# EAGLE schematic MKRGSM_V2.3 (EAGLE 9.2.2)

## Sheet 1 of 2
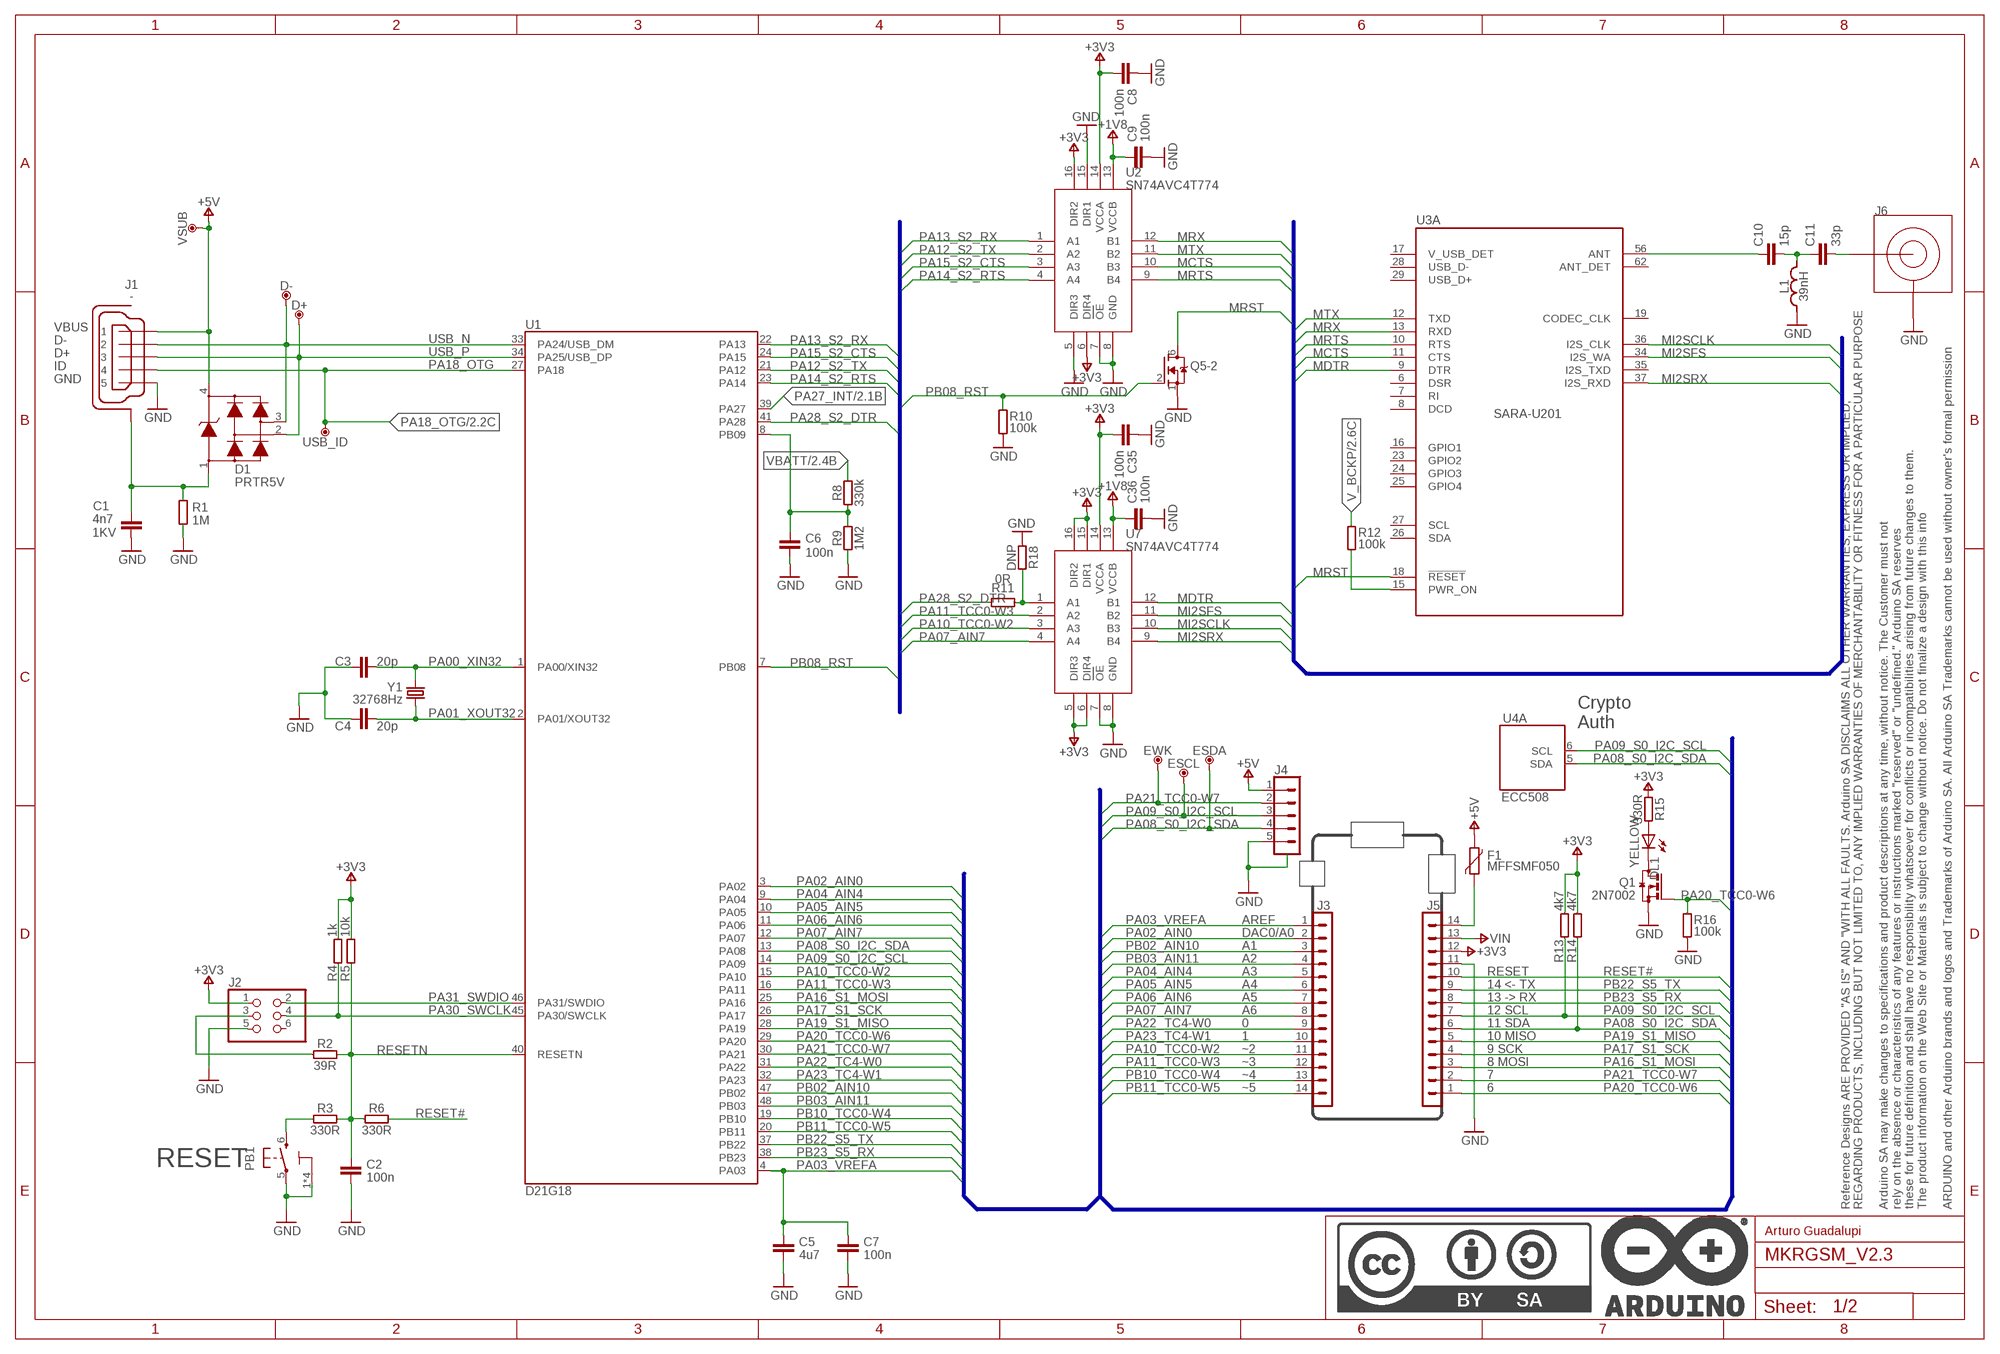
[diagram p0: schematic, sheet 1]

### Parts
C1  4n7  C4.7NF-0805  [0805-R2013X50N]
C2  100n  C-100NF-0402  [0402-1005X55N]
C3  20p  C-20PF-0402  [0402-1005X55N]
C4  20p  C-20PF-0402  [0402-1005X55N]
C5  4u7  C-4.7UF-0402  [0402-1005X55N]
C6  100n  C-100NF-0402  [0402-1005X55N]
C7  100n  C-100NF-0402  [0402-1005X55N]
C8  100n  C-100NF-0402  [0402-1005X55N]
C9  100n  C-100NF-0402  [0402-1005X55N]
C10  15p  C-15PF-0402  [0402-1005X55N]
C11  33p  C-33PF-0402  [0402-1005X55N]
C35  100n  C-100NF-0402  [0402-1005X55N]
C36  100n  C-100NF-0402  [0402-1005X55N]
D1  PRTR5V  PRTR5V0U2X,215  [SOT190P230X110-4N]
D+  DNP  TPTP-1.00MM  [TP-1.00MM]
D-  DNP  TPTP-1.00MM  [TP-1.00MM]
DL1  YELLOW  LED-YELLOW-0603  [LEDC1608X80N-AK]
ESCL  DNP  TPTP-1.00MM  [TP-1.00MM]
ESDA  DNP  TPTP-1.00MM  [TP-1.00MM]
EWK  DNP  TPTP-1.00MM  [TP-1.00MM]
F1  MFFSMF050  PTC  [0603-1608X90N]
FRAME1  DNP  A3-FRAME  [FRAME]
J1  -  USB-MICRO  [ZX62-AB-5PA]
J2  DNP  PINHD-2X03-DNPSMD-NH  [2X3_SMT]
J3  -  PINHD-1X14-SM-MALE/FEMALETH-SMD  [1X14_SMD_TH]
J4  -  SM05B-SRSS-TB  [SM05B-SRSS-TB]
J5  -  PINHD-1X14-SM-MALE/FEMALETH-SMD  [1X14_SMD_TH]
J6  -  UFL  [U.FL-R-SMT-1(60)]
L1  39nH  L-39NH-0402  [C0402]
PB1  PTS820  TACTILE1PTS820-NH  [C&K_PTS820_NO_HOLES]
Q1  2N7002  2N7002T  [SOTFL50P160X78-3]
Q5  2N7002DW-7-FNO_PAD  [PWR_SC70-6L2]
R1  1M  R-1M-0402  [0402-1005X55N]
R2  39R  R-39R-0402  [0402-1005X55N]
R3  330R  R-330R-0402  [0402-1005X55N]
R4  1k  R-1K-0402  [0402-1005X55N]
R5  10k  R-10K-0402  [0402-1005X55N]
R6  330R  R-330R-0402  [0402-1005X55N]
R8  330k  R-330K-0402  [0402-1005X55N]
R9  1M2  R-1M2-0402  [0402-1005X55N]
R10  100k  R-100K-0402  [0402-1005X55N]
R11  0R  R-0R-0402  [0402-1005X55N]
R12  100k  R-100K-0402  [0402-1005X55N]
R13  4k7  R-4K7-0402  [0402-1005X55N]
R14  4k7  R-4K7-0402  [0402-1005X55N]
R15  330R  R-330R-0402  [0402-1005X55N]
R16  100k  R-100K-0402  [0402-1005X55N]
R18  DNP  R-DNP-0402  [0402-1005X55N]
U1  D21G18  ATSAMD21G18A-48QFN  [QFN50P700X700X90-49XN-EPSQ515]
U2  SN74AVC4T774  [RSV]
U3  SARA-U201  SARA-U2  [SARA-96]
U4  ECC508  ATECC508A-MAHDA-T8-UDFN  [SON50P300X200X60-9N-EP160X140]
U7  SN74AVC4T774  [RSV]
USB_ID  DNP  TPTP-1.00MM  [TP-1.00MM]
VSUB  DNP  TPTP-1.00MM  [TP-1.00MM]
Y1  32768Hz  32.768KHZ  [ABS07]

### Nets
+1V8: C9.1 C36.1 U2.13(VCCB) U7.13(VCCB) ; also sheet 2
+3V3: C8.2 C35.2 J2.1 J5.12 R4.2 R5.2 R13.2 R14.2 R15.1 U2.6(DIR4) U2.14(VCCA) U2.16(DIR2) U7.5(DIR3) U7.6(DIR4) U7.14(VCCA) U7.15(DIR1) U7.16(DIR2) ; also sheet 2
+5V: D1.4 F1.2 J1.1 J4.1 VSUB.X ; also sheet 2
GND: C1.2 C2.2 C3.1 C4.1 C5.2 C6.2 C7.2 C8.1 C9.2 C35.1 C36.2 J1.5 J2.5 J4.5 J4.SH1(SH) J4.SH2(SH) J5.11 J6.GND1(GND) J6.GND2(GND) L1.1 PB1.1 PB1.2 PB1.3 PB1.4 PB1.5 Q1.S Q5.1(-2:S) R1.1 R9.1 R10.1 R16.1 R18.1 U2.5(DIR3) U2.7(OE) U2.8(GND) U2.15(DIR1) U7.7(OE) U7.8(GND) ; also sheet 2
MCTS: U2.10(B3) U3.11(A:CTS)
MDTR: U3.9(A:DTR) U7.12(B1)
MI2SCLK: U3.36(A:I2S_CLK) U7.10(B3)
MI2SFS: U3.34(A:I2S_WA) U7.11(B2)
MI2SRX: U3.37(A:I2S_RXD) U7.9(B4)
MRST: Q5.6(-2:D) U3.18(A:!RESET)
MRTS: U2.9(B4) U3.10(A:RTS)
MRX: U2.12(B1) U3.13(A:RXD)
MTX: U2.11(B2) U3.12(A:TXD)
N17658775: PB1.6 R3.1
N$1: C1.1 D1.1 J1.6(SH) J1.7(SH) J1.8(SH) J1.9(SH) J1.10(SH) J1.11(SH) R1.2
N$2: F1.1 J5.14
N$4: J2.3 R2.1
N$5: C10.1 U3.56(A:ANT)
N$6: C6.1 R8.1 R9.2 U1.8(PB09)
N$7: DL1.A R15.2
N$8: C11.2 J6.SIG
N$9: R11.1 R18.2 U7.1(A1)
N$10: DL1.C Q1.D
N$13: R12.1 U3.15(A:PWR_ON)
N$14: C10.2 C11.1 L1.2
PA00_XIN32: C3.2 U1.1(PA00/XIN32) Y1.2
PA01_XOUT32: C4.2 U1.2(PA01/XOUT32) Y1.1
PA02_AIN0: J3.2 U1.3(PA02)
PA03_VREFA: C5.1 C7.1 J3.1 U1.4(PA03)
PA04_AIN4: J3.5 U1.9(PA04)
PA05_AIN5: J3.6 U1.10(PA05)
PA06_AIN6: J3.7 U1.11(PA06)
PA07_AIN7: J3.8 U1.12(PA07) U7.4(A4)
PA08_S0_I2C_SDA: ESDA.X J4.4 J5.6 R14.1 U1.13(PA08) U4.5(A:SDA) ; also sheet 2
PA09_S0_I2C_SCL: ESCL.X J4.3 J5.7 R13.1 U1.14(PA09) U4.6(A:SCL) ; also sheet 2
PA10_TCC0-W2: J3.11 U1.15(PA10) U7.3(A3)
PA11_TCC0-W3: J3.12 U1.16(PA11) U7.2(A2)
PA12_S2_TX: U1.21(PA12) U2.2(A2)
PA13_S2_RX: U1.22(PA13) U2.1(A1)
PA14_S2_RTS: U1.23(PA14) U2.4(A4)
PA15_S2_CTS: U1.24(PA15) U2.3(A3)
PA16_S1_MOSI: J5.3 U1.25(PA16)
PA17_S1_SCK: J5.4 U1.26(PA17)
PA18_OTG: J1.4 U1.27(PA18) USB_ID.X ; also sheet 2
PA19_S1_MISO: J5.5 U1.28(PA19)
PA20_TCC0-W6: J5.1 Q1.G R16.2 U1.29(PA20)
PA21_TCC0-W7: EWK.X J4.2 J5.2 U1.30(PA21)
PA22_TC4-W0: J3.9 U1.31(PA22)
PA23_TC4-W1: J3.10 U1.32(PA23)
PA27_INT: U1.39(PA27) ; also sheet 2
PA28_S2_DTR: R11.2 U1.41(PA28)
PA30_SWCLK: J2.4 R4.1 U1.45(PA30/SWCLK)
PA31_SWDIO: J2.2 U1.46(PA31/SWDIO)
PB02_AIN10: J3.3 U1.47(PB02)
PB03_AIN11: J3.4 U1.48(PB03)
PB08_RST: Q5.2(-2:G) R10.2 U1.7(PB08)
PB10_TCC0-W4: J3.13 U1.19(PB10)
PB11_TCC0-W5: J3.14 U1.20(PB11)
PB22_S5_TX: J5.9 U1.37(PB22)
PB23_S5_RX: J5.8 U1.38(PB23)
RESET#: J5.10 R6.2
RESETN: C2.1 R2.2 R3.2 R5.1 R6.1 U1.40(RESETN)
USB_N [usb]: D1.3 D-.X J1.2 U1.33(PA24/USB_DM) ; also sheet 2
USB_P [usb]: D1.2 D+.X J1.3 U1.34(PA25/USB_DP) ; also sheet 2
V_BCKP: R12.2 ; also sheet 2
VBATT: R8.2 ; also sheet 2
VIN: J5.13 ; also sheet 2
Unconnected: J2.6 U3.6(A:DSR) U3.7(A:RI) U3.8(A:DCD) U3.16(A:GPIO1) U3.17(A:V_USB_DET) U3.19(A:CODEC_CLK) U3.23(A:GPIO2) U3.24(A:GPIO3) U3.25(A:GPIO4) U3.26(A:SDA) U3.27(A:SCL) U3.28(A:USB_D-) U3.29(A:USB_D+) U3.35(A:I2S_TXD) U3.62(A:ANT_DET)

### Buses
PA03_VREFA,PA02_AIN0,PB02_AIN10,PB03_AIN11,PA04_AIN4,PA05_AIN5,PA06_AIN6,PA07_AIN7,PA22_TC4-W0,PA23_TC4-W1,PA10_TCC0-W2,PA11_TCC0-W3,PB10_TCC0-W4,PB11_TCC0-W5,PA20_TCC0-W6,PA21_TCC0-W7,PA16_S1_MOSI,PA17_S1_SCK,PA19_S1_MISO,PA08_S0_I2C_SDA,PA09_S0_I2C_SCL,PB23_S5_RX,PB22_S5_TX,RESET#
MI2SCLK
B$2

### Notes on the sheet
- Crypto
  Auth
- AREF
- DAC0/A0
- A1
- A2
- A3 | RESET
- A4 | 14 <- TX
- A5 | 13 -> RX
- A6 | 12 SCL
- 0 | 11 SDA
- 1 | 10 MISO
- ~2 | 9 SCK
- ~3 | 8 MOSI
- ~4 | 7
- ~5 | 6
- RESET
- Arturo Guadalupi

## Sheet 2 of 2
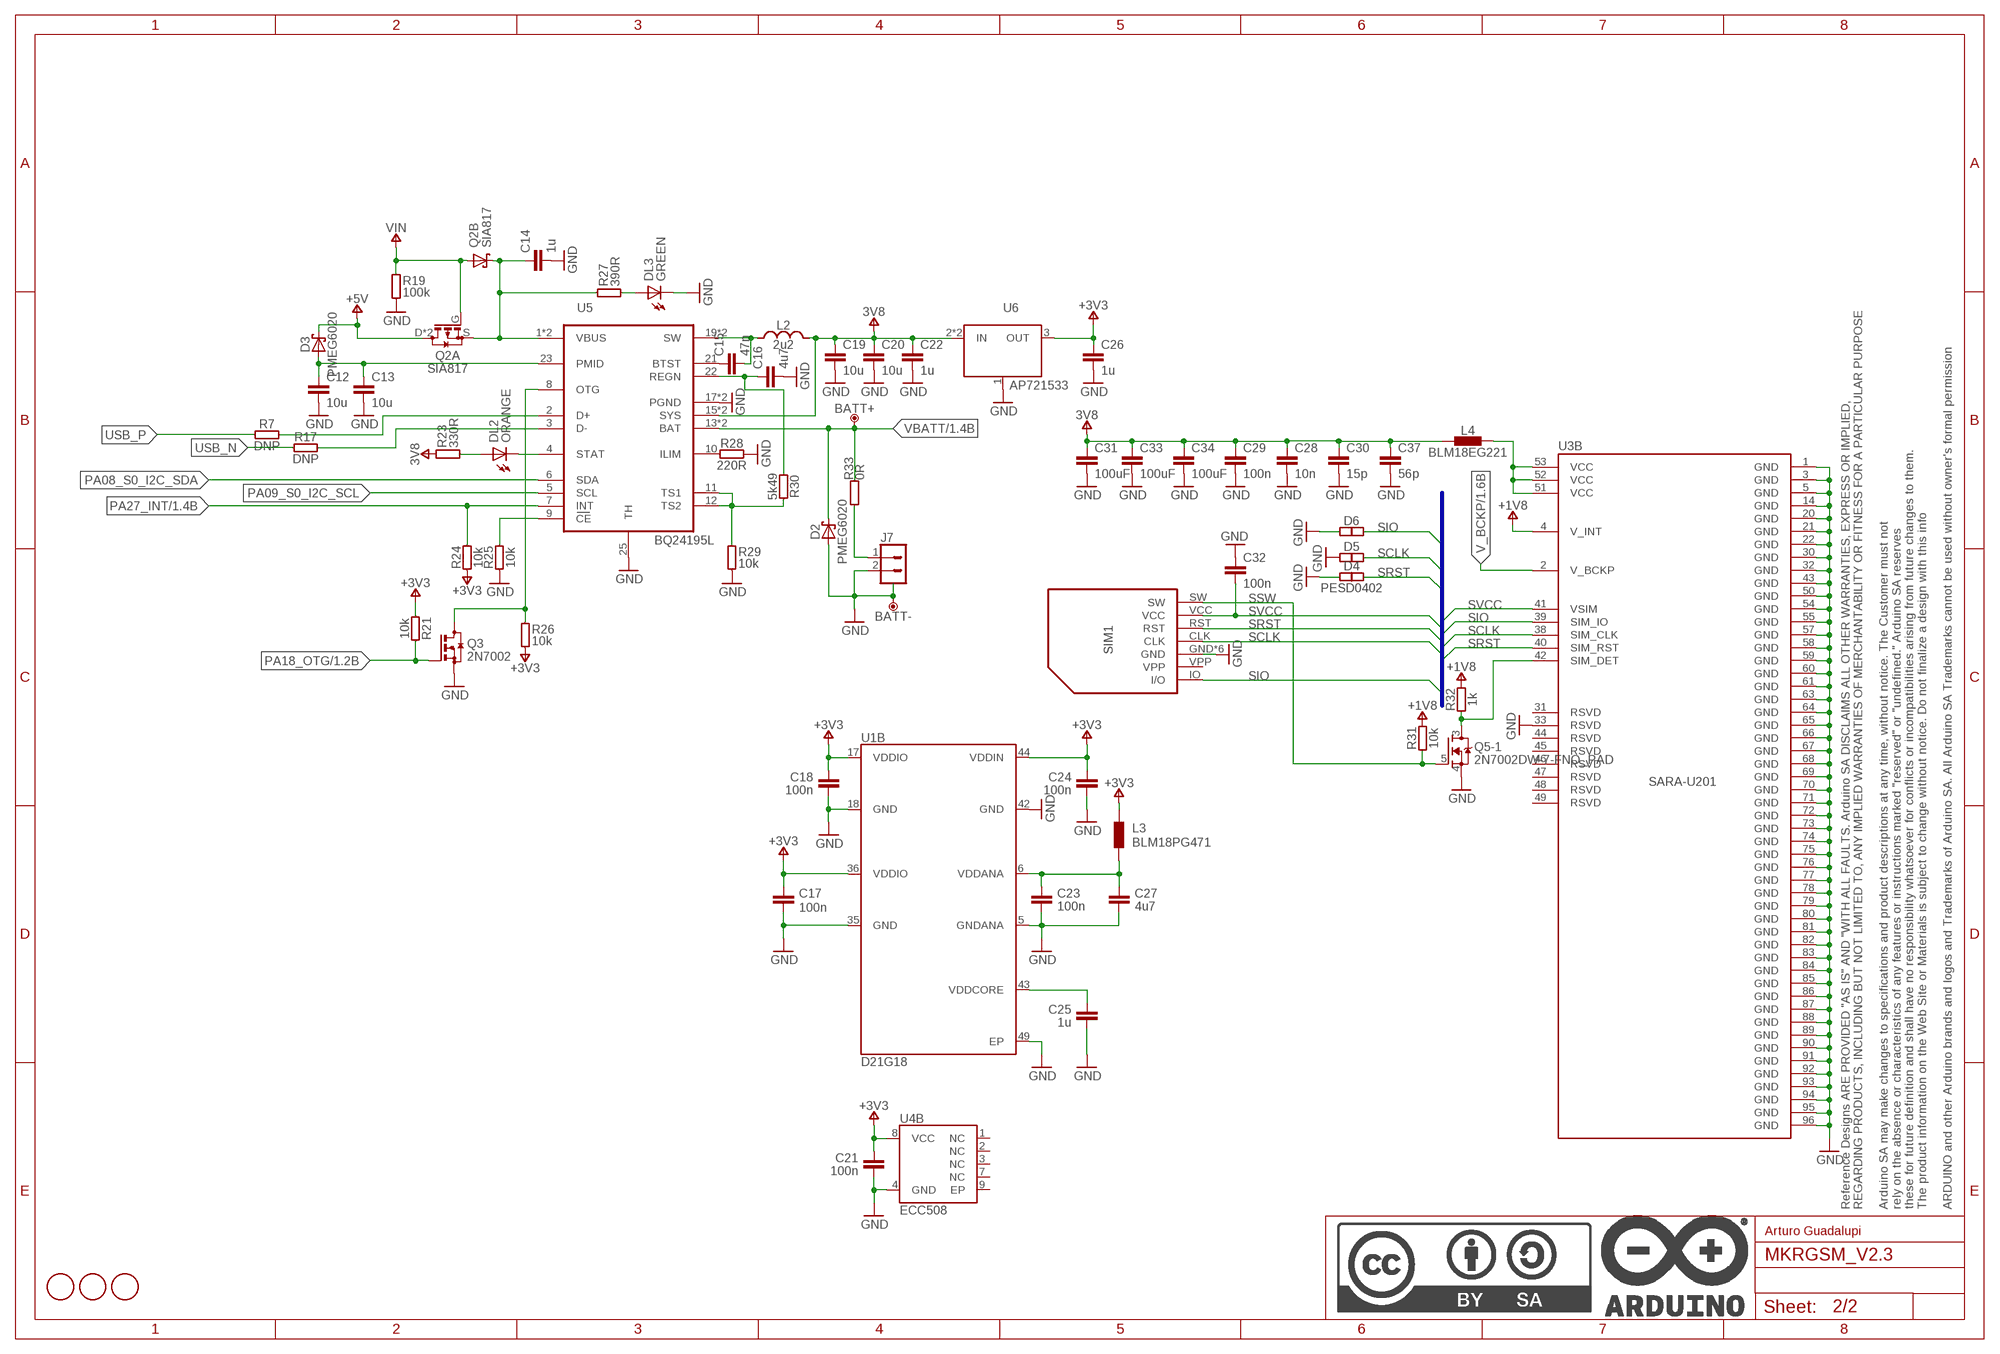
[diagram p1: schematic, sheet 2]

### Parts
BATT+  DNP  TPTP-1.00MM  [TP-1.00MM]
BATT-  DNP  TPTP-1.00MM  [TP-1.00MM]
C12  10u  C-10UF-0603  [0603-1608X90N]
C13  10u  C-10UF-0603  [0603-1608X90N]
C14  1u  C-1UF-0402  [0402-1005X55N]
C15  47n  C-47N-0402  [0402-1005X55N]
C16  4u7  C-4.7UF-0402  [0402-1005X55N]
C17  100n  C-100NF-0402  [0402-1005X55N]
C18  100n  C-100NF-0402  [0402-1005X55N]
C19  10u  C-10UF-0603  [0603-1608X90N]
C20  10u  C-10UF-0603  [0603-1608X90N]
C21  100n  C-100NF-0402  [0402-1005X55N]
C22  1u  C-1UF-0402  [0402-1005X55N]
C23  100n  C-100NF-0402  [0402-1005X55N]
C24  100n  C-100NF-0402  [0402-1005X55N]
C25  1u  C-1UF-0402  [0402-1005X55N]
C26  1u  C-1UF-0402  [0402-1005X55N]
C27  4u7  C-4.7UF-0603  [0603-1608X90N]
C28  10n  C-10NF-0402  [0402-1005X55N]
C29  100n  C-100NF-0402  [0402-1005X55N]
C30  15p  C-15PF-0402  [0402-1005X55N]
C31  100uF  C-100UF-1206  [C1206]
C32  100n  C-100NF-0402  [0402-1005X55N]
C33  100uF  C-100UF-1206  [C1206]
C34  100uF  C-100UF-1206  [C1206]
C37  56p  C-56P-0402  [0402-1005X55N]
D2  PMEG6020  PMEG6020AELRX  [SODFL3517X110N]
D3  PMEG6020  PMEG6020AELRX  [SODFL3517X110N]
D4  PESD0402  PESD  [0402-1005X55N]
D5  PESD0402  PESD  [0402-1005X55N]
D6  PESD0402  PESD  [0402-1005X55N]
DL2  ORANGE  LED-ORANGE-0603  [LEDC1608X80N-AK]
DL3  GREEN  LED-GREEN-0603  [LEDC1608X80N-AK]
FD1  DNP  FIDUCIAL-1.5MM  [FD-1-1.5]
FD2  DNP  FIDUCIAL-1.5MM  [FD-1-1.5]
FD3  DNP  FIDUCIAL-1.5MM  [FD-1-1.5]
FRAME2  DNP  A3-FRAME  [FRAME]
J7  -  BATTERY  [JST-S2B-PH-SM4-TB]
L2  2u2  LSRP  [SRP4020]
L3  BLM18PG471  FERRITE-470R  [0603-1608X90N]
L4  BLM18EG221  FERRITE-220R  [0603-1608X90N]
Q2  SIA817  SIA817EDJ  [SON65P205X205X75-8N-MWSD]
Q3  2N7002  2N7002T  [SOTFL50P160X78-3]
R7  DNP  R-DNP-0402  [0402-1005X55N]
R17  DNP  R-DNP-0402  [0402-1005X55N]
R19  100k  R-100K-0402  [0402-1005X55N]
R21  10k  R-10K-0402  [0402-1005X55N]
R23  330R  R-330R-0402  [0402-1005X55N]
R24  10k  R-10K-0402  [0402-1005X55N]
R25  10k  R-10K-0402  [0402-1005X55N]
R26  10k  R-10K-0402  [0402-1005X55N]
R27  390R  R-390R-0402  [0402-1005X55N]
R28  220R  R-220R-0402  [0402-1005X55N]
R29  10k  R-10K-0402  [0402-1005X55N]
R30  5k49  R-5K49-0402  [0402-1005X55N]
R31  10k  R-10K-0402  [0402-1005X55N]
R32  1k  R-1K-0402  [0402-1005X55N]
R33  0R  R-0R-0603  [C0603]
SIM1  -  SIM  [MICROSIM8]
U5  BQ24195L  BQ24195QFN-24  [QFN24]
U6  AP721533  AP7215-33YG  [SOT89-3L]

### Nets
+1V8: R31.2 R32.2 U3.4(B:V_INT) ; also sheet 1
+3V3: C17.1 C18.1 C21.1 C24.1 C26.1 L3.1 R21.1 R24.1 R26.1 U1.17(VDDIO) U1.36(VDDIO) U1.44(VDDIN) U4.8(B:VCC) U6.3(OUT) ; also sheet 1
+3V8: C19.1 C20.1 C22.1 C28.1 C29.1 C30.1 C31.1 C33.1 C34.1 C37.1 L2.2 L4.1 R23.2 U5.15(SYS) U5.16(SYS) U6.2(IN) U6.TH(IN) ; supply symbol labelled 3V8
+5V: D3.C Q2.D2(A:D) Q2.D(A:D) ; also sheet 1
GND: BATT-.X C12.2 C13.2 C14.2 C16.2 C17.2 C18.2 C19.2 C20.2 C21.2 C22.2 C23.2 C24.2 C25.2 C26.2 C27.2 C28.2 C29.2 C30.2 C31.2 C32.1 C33.2 C34.2 C37.2 D2.A D4.1 D5.1 D6.1 DL3.C J7.2 J7.3(SH) J7.4(SH) Q3.S Q5.4(-1:S) R19.1 R25.1 R28.2 R29.1 SIM1.GND SIM1.SH1(GND) SIM1.SH2(GND) SIM1.SH3(GND) SIM1.SH4(GND) SIM1.SH5(GND) U1.5(GNDANA) U1.18(GND) U1.35(GND) U1.42(GND) U1.49(EP) U3.1(B:GND) U3.3(B:GND) U3.5(B:GND) U3.14(B:GND) U3.20(B:GND) U3.21(B:GND) U3.22(B:GND) U3.30(B:GND) U3.32(B:GND) U3.33(B:RSVD) U3.43(B:GND) U3.50(B:GND) U3.54(B:GND) U3.55(B:GND) U3.57(B:GND) U3.58(B:GND) U3.59(B:GND) U3.60(B:GND) U3.61(B:GND) U3.63(B:GND) U3.64(B:GND) U3.65(B:GND) U3.66(B:GND) U3.67(B:GND) U3.68(B:GND) U3.69(B:GND) U3.70(B:GND) U3.71(B:GND) U3.72(B:GND) U3.73(B:GND) U3.74(B:GND) U3.75(B:GND) U3.76(B:GND) U3.77(B:GND) U3.78(B:GND) U3.79(B:GND) U3.80(B:GND) U3.81(B:GND) U3.82(B:GND) U3.83(B:GND) U3.84(B:GND) U3.85(B:GND) U3.86(B:GND) U3.87(B:GND) U3.88(B:GND) U3.89(B:GND) U3.90(B:GND) U3.91(B:GND) U3.92(B:GND) U3.93(B:GND) U3.94(B:GND) U3.95(B:GND) U3.96(B:GND) U4.4(B:GND) U5.17(PGND) U5.18(PGND) U5.25(TH) U6.1(GND/ADJ) ; also sheet 1
N17798864: DL2.A R23.1
N17834267: DL3.A R27.1
N17852357: C23.1 C27.1 L3.2 U1.6(VDDANA)
N17852431: C25.1 U1.43(VDDCORE)
N$3: J7.1 R33.1
N$11: Q5.3(-1:D) R32.1 U3.42(B:SIM_DET)
N$12: L4.2 U3.51(B:VCC) U3.52(B:VCC) U3.53(B:VCC)
N$15: C15.2 L2.1 U5.19(SW) U5.20(SW)
N$16: R7.2 U5.2(D+)
N$17: C14.1 Q2.K2(B:C) Q2.K(B:C) Q2.S(A:S) R27.2 U5.1(VBUS) U5.24(VBUS)
N$18: C15.1 U5.21(BTST)
N$19: R28.1 U5.10(ILIM)
N$20: R17.2 U5.3(D-)
N$21: C16.1 R30.1 U5.22(REGN)
N$22: Q3.D R26.2 U5.8(OTG)
N$23: R29.2 R30.2 U5.11(TS1) U5.12(TS2)
N$24: R25.2 U5.9(CE)
PA08_S0_I2C_SDA: U5.6(SDA) ; also sheet 1
PA09_S0_I2C_SCL: U5.5(SCL) ; also sheet 1
PA18_OTG: Q3.G R21.2 ; also sheet 1
PA27_INT: R24.2 U5.7(INT) ; also sheet 1
SCLK: D5.2 SIM1.CLK U3.38(B:SIM_CLK)
SIO: D6.2 SIM1.IO(I/O) U3.39(B:SIM_IO)
SRST: D4.2 SIM1.RST U3.40(B:SIM_RST)
SSW: Q5.5(-1:G) R31.1 SIM1.SW
STAT: DL2.C U5.4(STAT)
SVCC: C32.2 SIM1.VCC U3.41(B:VSIM)
USB_N [usb]: R17.1 ; also sheet 1
USB_P [usb]: R7.1 ; also sheet 1
V_BCKP: U3.2(B:V_BCKP) ; also sheet 1
VBATT: BATT+.X D2.C R33.2 U5.13(BAT) U5.14(BAT) ; also sheet 1
VIN: Q2.A(B:A) Q2.G(A:G) R19.2 ; also sheet 1
VUSB1: C12.1 C13.1 D3.A U5.23(PMID)
Unconnected: SIM1.VPP U3.31(B:RSVD) U3.44(B:RSVD) U3.45(B:RSVD) U3.46(B:RSVD) U3.47(B:RSVD) U3.48(B:RSVD) U3.49(B:RSVD) U4.1(B:NC) U4.2(B:NC) U4.3(B:NC) U4.7(B:NC) U4.9(B:EP)

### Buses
B$1

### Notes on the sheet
- Arturo Guadalupi

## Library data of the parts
BATT+ BATT- D+ D- ESCL ESDA EWK USB_ID VSUB = Arduino-utility:TP: Testpoint; DATASHEET: DNP; DISTRIBUTOR-LINK: DNP; DISTRIBUTOR-PN: DNP; MANUFACTURER: DNP; MANUFACTURER-PN: DNP
C1 = Arduino-rcl:C: SMD Capacitor; CODE-ARDUINO: 0689; DATASHEET: http://www.kemet.com/Lists/ProductCatalog/Attachments/40/KEM_C1010_X7R_HV_SMD.pdf; DISTRIBUTOR-LINK: www.kemet.com/docfinder?Partnumber=C0805C472KDRACTU; DISTRIBUTOR-PN: 399-6738-1-ND; MANUFACTURER: Kemet; MANUFACTURER-PN: C0805C472KDRACTU; NOTE: -; VOLTAGE: 1KV
C2 C6-C9 C17 C18 C21 C23 C24 C29 C32 C35 C36 = Arduino-rcl:C: SMD Capacitor; CODE-ARDUINO: 0132; DATASHEET: http://www.tdk.com/pdf/TDKMLCCCapRange.pdf; DISTRIBUTOR-LINK: http://www.digikey.com/product-detail/en/tdk-corporation/C1005X5R1H104K050BB/445-5942-1-ND/2443982; DISTRIBUTOR-PN: 445-5942-1-ND; MANUFACTURER: TDK; MANUFACTURER-PN: C1005X5R1H104K050BB; NOTE: -
C3 C4 = Arduino-rcl:C: SMD Capacitor; CODE-ARDUINO: 2188; DATASHEET: http://www.kemet.com/docfinder?Partnumber=CBR04C200J5GAC; DISTRIBUTOR-LINK: http://www.digikey.com/product-detail/en/kemet/CBR04C200J5GAC/399-6173-1-ND/2732143; DISTRIBUTOR-PN: 399-6173-1-ND; MANUFACTURER: Kemet; MANUFACTURER-PN: CBR04C200J5GAC; NOTE: -
C5 C16 = Arduino-rcl:C: SMD Capacitor; CODE-ARDUINO: 0833; DATASHEET: http://search.murata.co.jp/Ceramy/image/img/A01X/partnumbering_e_01.pdf; DISTRIBUTOR-LINK: http://www.digikey.com/product-detail/en/murata-electronics-north-america/GRM155R60J475ME47D/490-5915-1-ND/3719860; DISTRIBUTOR-PN: 490-5915-1-ND; MANUFACTURER: Murata; MANUFACTURER-PN: GRM155R60J475ME47D; NOTE: -
C10 C30 = Arduino-rcl:C: SMD Capacitor; CODE-ARDUINO: -; DATASHEET: http://search.murata.co.jp/Ceramy/image/img/A01X/partnumbering_e_01.pdf; DISTRIBUTOR-LINK: https://www.digikey.com/product-detail/en/murata-electronics-north-america/GRM1555C1H150JA01D/490-5888-1-ND/3315234; DISTRIBUTOR-PN: 490-5888-1-ND; MANUFACTURER: Murata; MANUFACTURER-PN: GRM1555C1H150JA01D; NOTE: -
C11 = Arduino-rcl:C: SMD Capacitor; CODE-ARDUINO: -; DATASHEET: http://www.murata.com/~/media/webrenewal/support/library/catalog/products/capacitor/mlcc/c02e.pdf; DISTRIBUTOR-LINK: http://www.digikey.com/product-search/en?keywords=490-5936-1-ND; DISTRIBUTOR-PN: 490-5936-1-ND; MANUFACTURER: Murata; MANUFACTURER-PN: GRM1555C1H330JA01D; NOTE: -
C12 C13 C19 C20 = Arduino-rcl:C: SMD Capacitor; CODE-ARDUINO: 2213; DATASHEET: http://www.murata.com/~/media/webrenewal/support/library/catalog/products/capacitor/mlcc/c02e.pdf; DISTRIBUTOR-LINK: http://www.digikey.com/product-search/en?keywords=490-10728-1-ND; DISTRIBUTOR-PN: 490-10728-1-ND; MANUFACTURER: Murata; MANUFACTURER-PN: GRM188R61C106KAALD; NOTE: -
C14 C22 C25 C26 = Arduino-rcl:C: SMD Capacitor; CODE-ARDUINO: 0133; DATASHEET: http://search.murata.co.jp/Ceramy/image/img/A01X/partnumbering_e_01.pdf; DISTRIBUTOR-LINK: http://www.digikey.com/product-detail/en/murata-electronics-north-america/GRM155R61E105KA12D/490-10017-1-ND/5026367; DISTRIBUTOR-PN: 490-10017-1-ND; MANUFACTURER: Murata; MANUFACTURER-PN: GRM155R61E105KA12D; NOTE: -
C15 = Arduino-rcl:C: SMD Capacitor; CODE-ARDUINO: 2216; DATASHEET: http://www.murata.com/~/media/webrenewal/support/library/catalog/products/capacitor/mlcc/c02e.pdf; DISTRIBUTOR-LINK: https://www.digikey.com/product-detail/en/murata-electronics-north-america/GRM155R71E473KA88D/490-3254-1-ND/702795; DISTRIBUTOR-PN: 490-3254-1-ND; MANUFACTURER: Murata; MANUFACTURER-PN: GRM155R71E473KA88D; NOTE: -
C27 = Arduino-rcl:C: SMD Capacitor; CODE-ARDUINO: 0458; DATASHEET: http://www.murata.com/~/media/webrenewal/support/library/catalog/products/capacitor/mlcc/c02e.pdf; DISTRIBUTOR-LINK: http://www.digikey.com/product-search/en?keywords=490-7203-1-ND; DISTRIBUTOR-PN: 490-7203-1-ND; MANUFACTURER: Murata; MANUFACTURER-PN: GRM188R61E475KE11D; NOTE: -
C28 = Arduino-rcl:C: SMD Capacitor; CODE-ARDUINO: 0165; DATASHEET: http://search.murata.co.jp/Ceramy/image/img/A01X/partnumbering_e_01.pdf; DISTRIBUTOR-LINK: http://www.digikey.com/product-detail/en/murata-electronics-north-america/GRM155R71H103KA88J/490-6351-1-ND/3845548; DISTRIBUTOR-PN: 490-6351-1-ND; MANUFACTURER: Murata; MANUFACTURER-PN: GRM155R71H103KA88J; NOTE: -
C31 C33 C34 = Arduino-rcl:C: SMD Capacitor; CODE-ARDUINO: -; DATASHEET: http://search.murata.co.jp/Ceramy/image/img/A01X/partnumbering_e_01.pdf; DISTRIBUTOR-LINK: https://www.digikey.com/product-detail/en/murata-electronics-north-america/GRM31CD80J107ME39L/490-10525-1-ND/5026461; DISTRIBUTOR-PN: 490-10525-1-ND; MANUFACTURER: Murata; MANUFACTURER-PN: GRM31CD80J107ME39L; NOTE: -
C37 = Arduino-rcl:C: SMD Capacitor; CODE-ARDUINO: -; DATASHEET: http://www.mouser.com/ds/2/281/c02e-2905.pdf; DISTRIBUTOR-LINK: http://www.mouser.it/ProductDetail/Murata-Electronics/GRM1555C1E560JA01D/?qs=sGAEpiMZZMs0AnBnWHyRQA3eyUP2RfX77sTVhhB4SFb8UyJFwKUI8g%3d%3d; DISTRIBUTOR-PN: 81-GRM1555C1E560JA1D; MANUFACTURER: Murata; MANUFACTURER-PN: GRM1555C1E560JA01D; NOTE: -
D1 = Arduino-diodes:PRTR5V0U2X,215: USB ESD protection; DATASHEET: http://www.nxp.com/documents/data_sheet/PRTR5V0U2X.pdf; DISTRIBUTOR-LINK: http://www.digikey.com/product-detail/en/nxp-semiconductors/PRTR5V0U2X,215/568-4140-1-ND/1589981; DISTRIBUTOR-PN: 568-4140-1-ND; MANUFACTURER: NXP; MANUFACTURER-PN: PRTR5V0U2X,215
D2 D3 = Arduino-diodes:PMEG6020AELRX: 60 V, 2 A low leakage current Schottky barrier rectifier; DATASHEET: http://www.nxp.com/documents/data_sheet/PMEG6020AELR.pdf; DISTRIBUTOR-LINK: http://www.digikey.com/products/en?keywords=%20568-12710-1-ND; DISTRIBUTOR-PN: 568-12710-1-ND; MANUFACTURER: NXP; MANUFACTURER-PN: PMEG6020AELRX
D4-D6 = Arduino-diodes:PESD; DATASHEET: http://www.littelfuse.com/~/media/electronics/product_specifications/polymer_esd_suppressors/littelfuse_polymer_esd_suppressor_pesd0402_140_product_specification.pdf.pdf; DISTRIBUTOR-LINK: https://www.digikey.com/product-detail/en/littelfuse-inc/PESD0402-140/PESD0402-140CT-ND/1968526; DISTRIBUTOR-PN: PESD0402-140CT-ND; MANUFACTURER: Littlefuse; MANUFACTURER-PN: PESD0402-140
DL1 = Arduino-diodes:LED: LED; DATASHEET: http://media.digikey.com/pdf/Data%20Sheets/Avago%20PDFs/HSMz-Czzz.pdf; DISTRIBUTOR-LINK: http://www.digikey.com/product-detail/en/broadcom-limited/HSMY-C190/516-1424-1-ND/637748; DISTRIBUTOR-PN: 516-1424-1-ND; MANUFACTURER: Avago; MANUFACTURER-PN: HSMY-C190
DL2 = Arduino-diodes:LED: LED; DATASHEET: http://media.digikey.com/pdf/Data%20Sheets/Avago%20PDFs/HSMz-Czzz.pdf; DISTRIBUTOR-LINK: http://www.digikey.com/product-detail/en/broadcom-limited/HSMD-C190/516-2489-1-ND/2744915; DISTRIBUTOR-PN: 516-2489-1-ND; MANUFACTURER: Avago; MANUFACTURER-PN: HSMD-C190
DL3 = Arduino-diodes:LED: LED; DATASHEET: http://media.digikey.com/pdf/Data%20Sheets/Avago%20PDFs/HSMz-Czzz.pdf; DISTRIBUTOR-LINK: http://www.digikey.com/product-detail/en/broadcom-limited/HSMG-C190/516-1425-1-ND/637749; DISTRIBUTOR-PN: 516-1425-1-ND; MANUFACTURER: Avago; MANUFACTURER-PN: HSMG-C190
F1 = Arduino-rcl:PTC: SMD PTC; DATASHEET: http://www.bourns.com/docs/Product-Datasheets/mffsmf.pdf; DISTRIBUTOR-LINK: http://www.digikey.com/product-detail/en/bourns-inc/MF-FSMF050X-2/MF-FSMF050X-2CT-ND/2039389; DISTRIBUTOR-PN: MF-FSMF050X-2CT-ND; MANUFACTURER: Bourns Inc; MANUFACTURER-PN: MF-FSMF050X-2
FD1-FD3 = Arduino-utility:FIDUCIAL: Fiducial mount; DATASHEET: DNP; DISTRIBUTOR-LINK: DNP; DISTRIBUTOR-PN: DNP; MANUFACTURER: DNP; MANUFACTURER-PN: DNP
FRAME1 FRAME2 = Arduino-utility:A3-FRAME; CODE-ARDUINO: DNP; DATASHEET: DNP; DISTRIBUTOR-LINK: DNP; DISTRIBUTOR-PN: DNP; MANUFACTURER: DNP; MANUFACTURER-PN: DNP; NOTE: DNP
J1 = Arduino-connectors:USB-MICRO: USB - micro AB USB 2.0 Receptacle Connector 5 Position Surface Mount, Right Angle, Horizontal; DATASHEET: https://www.hirose.com/product/en/download_file/key_name/ZX/category/Catalog/doc_file_id/31704/?file_category_id=4&item_id=13&is_series=1; DISTRIBUTOR-LINK: http://www.digikey.com/product-detail/en/hirose-electric-co-ltd/ZX62-AB-5PA(31)/H125279CT-ND/5994741; DISTRIBUTOR-PN: H125279CT-ND; MANUFACTURER: Hirose; MANUFACTURER-PN: ZX62-AB-5PA(31)
J2 = Arduino-connectors:PINHD-2X03: PIN HEADER; DATASHEET: DNP; DISTRIBUTOR-LINK: DNP; DISTRIBUTOR-PN: DNP; MANUFACTURER: DNP; MANUFACTURER-PN: DNP
J3 J5 = Arduino-connectors:PINHD-1X14-SM: PIN HEADER; DATASHEET: -; DISTRIBUTOR-LINK: -; DISTRIBUTOR-PN: -; MANUFACTURER: ELDECO; MANUFACTURER-PN: FH254114DF08500T
J4 = Arduino-connectors:SM05B-SRSS-TB: CONN HEADER SH 5POS SIDE 1MM TIN Datasheet; DATASHEET: http://www.jst-mfg.com/product/pdf/eng/eSH.pdf; DISTRIBUTOR-LINK: http://www.digikey.com/product-detail/en/jst-sales-america-inc/SM05B-SRSS-TB(LF)(SN)/455-1805-1-ND/926876; DISTRIBUTOR-PN: 455-1805-1-ND; MANUFACTURER: JST; MANUFACTURER-PN: SM05B-SRSS-TB
J6 = Arduino-connectors:UFL: U.FL, Ultra Miniature Coaxial Connector Receptacle, Male Pin 50 Ohm Surface Mount Solder; DATASHEET: http://media.digikey.com/pdf/Data%20Sheets/Hirose%20PDFs/UFL%20Series.pdf; DISTRIBUTOR-LINK: http://www.digikey.com/product-search/en?keywords=U.FL-R-SMT-1(60); DISTRIBUTOR-PN: U.FL-R-SMT-1(60)-ND; MANUFACTURER: Hirose; MANUFACTURER-PN: U.FL-R-SMT-1(60)
J7 = Arduino-connectors:BATTERY: CONN HEADER PH SIDE 2POS 2MM SMD; DATASHEET: http://www.jst-mfg.com/product/pdf/eng/ePH.pdf; DISTRIBUTOR-LINK: http://www.digikey.com/product-detail/en/jst-sales-america-inc/S2B-PH-SM4-TB%28LF%29%28SN%29/455-1749-1-ND/926846; DISTRIBUTOR-PN: 455-1749-1-ND; MANUFACTURER: JST; MANUFACTURER-PN: S2B-PH-SM4-TB(LF)(SN)
L1 = Arduino-rcl:L: Inductors; CODE-ARDUINO: -; DATASHEET: http://search.murata.co.jp/Ceramy/image/img/P02/JELF243B-0009.pdf; DISTRIBUTOR-LINK: https://www.digikey.com/product-detail/en/murata-electronics-north-america/LQG15HN39NJ02D/490-1092-1-ND/584538; DISTRIBUTOR-PN: 490-1092-1-ND; MANUFACTURER: Murata; MANUFACTURER-PN: LQG15HN39NJ02D
L2 = Arduino-rcl:L: Inductors; CODE-ARDUINO: 2218; DATASHEET: http://www.bourns.com/docs/Product-Datasheets/SRP4020TA.pdf; DISTRIBUTOR-LINK: https://www.digikey.com/product-detail/en/bourns-inc/SRP4020TA-2R2M/SRP4020TA-2R2MCT-ND/4901068; DISTRIBUTOR-PN: SRP4020TA-2R2MCT-ND; MANUFACTURER: Bourns; MANUFACTURER-PN: SRP4020TA-2R2M
L3 = Arduino-rcl:FERRITE: SMD ferrite; DATASHEET: http://search.murata.co.jp/Ceramy/image/img/PDF/ENG/L0110S0100BLM18P.pdf; DISTRIBUTOR-LINK: http://www.digikey.com/product-detail/en/murata-electronics-north-america/BLM18PG471SN1D/490-5223-1-ND/1948399; DISTRIBUTOR-PN: 490-5223-1-ND; MANUFACTURER: Murata; MANUFACTURER-PN: BLM18PG471SN1D
L4 = Arduino-rcl:FERRITE: SMD ferrite; DATASHEET: http://www.murata.com/en-us/products/productdata/8796747366430/ENFA0021.pdf; DISTRIBUTOR-LINK: https://www.digikey.com/product-detail/en/murata-electronics-north-america/BLM18EG221SN1D/490-3992-1-ND/1016252; DISTRIBUTOR-PN: 490-3992-1-ND; MANUFACTURER: Murata; MANUFACTURER-PN: BLM18EG221SN1D
PB1 = Arduino-pushbuttons:TACTILE1: Tactile Switch SPST-NO Top Actuated Surface Mount; DATASHEET: http://www.ckswitches.com/media/1474/pts820.pdf; DISTRIBUTOR-LINK: https://www.digikey.com/product-detail/en/c-k/PTS820-J15M-SMTR-LFS/CKN10506CT-ND/4176681; DISTRIBUTOR-PN: PTS820 J25K SMTR LFS-ND; MANUFACTURER: C&K; MANUFACTURER-PN: PTS820 J25K SMTR LFS
Q1 Q3 = Arduino-transistors:2N7002T: MOSFET N-CH 60V 115MA SOT-523; DATASHEET: http://www.diodes.com/_files/datasheets/ds30301.pdf; DISTRIBUTOR-LINK: http://www.digikey.com/product-detail/en/diodes-incorporated/2N7002T-7-F/2N7002T-FDICT-ND/815290; DISTRIBUTOR-PN: 2N7002T-FDICT-ND; MANUFACTURER: Diodes Incorporated; MANUFACTURER-PN: 2N7002T-7-F
Q2 = Arduino-transistors:SIA817EDJ: MOSFET P-CH 30V 4.5A SC-70-6; DATASHEET: http://www.vishay.com/docs/62820/sia817edj.pdf; DISTRIBUTOR-LINK: http://www.digikey.com/product-detail/en/vishay-siliconix/SIA817EDJ-T1-GE3/SIA817EDJ-T1-GE3CT-ND/4142098; DISTRIBUTOR-PN: SIA817EDJ-T1-GE3CT-ND; MANUFACTURER: Vishay; MANUFACTURER-PN: SIA817EDJ-T1-GE3
Q5 = Arduino-transistors:2N7002DW-7-F: MOSFET 2N-CH 60V 0.23A SOT-363; DATASHEET: http://www.diodes.com/_files/datasheets/ds30120.pdf; DISTRIBUTOR-LINK: http://www.digikey.com/product-detail/en/diodes-incorporated/2N7002DW-7-F/2N7002DW-FDITR-ND/749948; DISTRIBUTOR-PN: 2N7002DW-FDITR-ND; MANUFACTURER: Diodes Incorporated; MANUFACTURER-PN: 2N7002DW-7-F
R1 = Arduino-rcl:R: SMD Resistor; CODE-ARDUINO: 0139; DATASHEET: www.yageo.com.tw/exep/pages/download/literatures/PYu-R_INT-thick_7.pdf; DISTRIBUTOR-LINK: http://www.digikey.com/product-detail/en/yageo/RC0402JR-07330RL/311-330JRCT-ND/729412; DISTRIBUTOR-PN: 311-330JRCT-ND; MANUFACTURER: Yageo; MANUFACTURER-PN: RC0402JR-07330RL; NOTE: NO
R2 = Arduino-rcl:R: SMD Resistor; CODE-ARDUINO: 0138; DATASHEET: www.yageo.com.tw/exep/pages/download/literatures/PYu-R_INT-thick_7.pdf; DISTRIBUTOR-LINK: http://www.digikey.com/product-detail/en/yageo/RC0402FR-0739RL/311-39.0LRCT-ND/729549; DISTRIBUTOR-PN: 311-39.0LRCT-ND; MANUFACTURER: Yageo; MANUFACTURER-PN: RC0402FR-0739RL; NOTE: NO
R3 R6 R15 R23 = Arduino-rcl:R: SMD Resistor; CODE-ARDUINO: 2229; DATASHEET: www.yageo.com.tw/exep/pages/download/literatures/PYu-R_INT-thick_7.pdf; DISTRIBUTOR-LINK: http://www.digikey.com/product-detail/en/yageo/RC0402FR-07330RL/311-330LRCT-ND/729541; DISTRIBUTOR-PN: 311-330LRCT-ND; MANUFACTURER: Yageo; MANUFACTURER-PN: RC0402FR-07330RL; NOTE: NO
R4 R32 = Arduino-rcl:R: SMD Resistor; CODE-ARDUINO: 0140; DATASHEET: www.yageo.com.tw/exep/pages/download/literatures/PYu-R_INT-thick_7.pdf; DISTRIBUTOR-LINK: http://www.digikey.com/product-detail/en/yageo/RC0402FR-071KL/311-1.00KLRCT-ND/729460; DISTRIBUTOR-PN: 311-1.00KLRCT-ND; MANUFACTURER: Yageo; MANUFACTURER-PN: RC0402FR-071KL; NOTE: NO
R5 R21 R24-R26 R29 R31 = Arduino-rcl:R: SMD Resistor; CODE-ARDUINO: 0136; DATASHEET: www.yageo.com.tw/exep/pages/download/literatures/PYu-R_INT-thick_7.pdf; DISTRIBUTOR-LINK: http://www.digikey.com/product-detail/en/yageo/RC0402FR-0710KL/311-10.0KLRCT-ND/729470; DISTRIBUTOR-PN: 311-10.0KLRCT-ND; MANUFACTURER: Yageo; MANUFACTURER-PN: RC0402FR-0710KL; NOTE: NO
R7 R17 R18 = Arduino-rcl:R: SMD Resistor; CODE-ARDUINO: DNP; DATASHEET: DNP; DISTRIBUTOR-LINK: DNP; DISTRIBUTOR-PN: DNP; MANUFACTURER: DNP; MANUFACTURER-PN: DNP; NOTE: NO
R8 = Arduino-rcl:R: SMD Resistor; CODE-ARDUINO: 2192; DATASHEET: www.yageo.com.tw/exep/pages/download/literatures/PYu-R_INT-thick_7.pdf; DISTRIBUTOR-LINK: http://www.digikey.com/product-detail/en/yageo/RC0402JR-07330KL/311-330KJRCT-ND/729413; DISTRIBUTOR-PN: 311-330KJRCT-ND; MANUFACTURER: Yageo; MANUFACTURER-PN: RC0402JR-07330KL; NOTE: NO
R9 = Arduino-rcl:R: SMD Resistor; CODE-ARDUINO: 2352; DATASHEET: www.yageo.com.tw/exep/pages/download/literatures/PYu-R_INT-thick_7.pdf; DISTRIBUTOR-LINK: http://www.digikey.com/products/en?keywords=RC0402FR-071M2L-ND; DISTRIBUTOR-PN: RC0402FR-071M2L-ND; MANUFACTURER: Yageo; MANUFACTURER-PN: RC0402FR-071M2L; NOTE: NO
R10 R12 R16 R19 = Arduino-rcl:R: SMD Resistor; CODE-ARDUINO: 0134; DATASHEET: www.yageo.com.tw/exep/pages/download/literatures/PYu-R_INT-thick_7.pdf; DISTRIBUTOR-LINK: http://www.digikey.com/product-detail/en/yageo/RC0402FR-07100KL/311-100KLRCT-ND/729473; DISTRIBUTOR-PN: 311-100KLRCT-ND; MANUFACTURER: Yageo; MANUFACTURER-PN: RC0402FR-07100KL; NOTE: NO
R11 = Arduino-rcl:R: SMD Resistor; CODE-ARDUINO: 0039; DATASHEET: www.yageo.com.tw/exep/pages/download/literatures/PYu-R_INT-thick_7.pdf; DISTRIBUTOR-LINK: http://www.digikey.com/product-detail/en/yageo/RC0402FR-070RL/311-0.0LRCT-ND/2827888; DISTRIBUTOR-PN: 311-0.0LRCT-ND; MANUFACTURER: Yageo; MANUFACTURER-PN: RC0402FR-070RL; NOTE: NO
R13 R14 = Arduino-rcl:R: SMD Resistor; CODE-ARDUINO: 2196; DATASHEET: www.yageo.com.tw/exep/pages/download/literatures/PYu-R_INT-thick_7.pdf; DISTRIBUTOR-LINK: http://www.digikey.com/product-detail/en/yageo/RC0402FR-074K7L/311-4.7KLRCT-ND/2827881; DISTRIBUTOR-PN: 311-4.7KLRCT-ND; MANUFACTURER: Yageo; MANUFACTURER-PN: RC0402FR-074K7L; NOTE: NO
R27 = Arduino-rcl:R: SMD Resistor; CODE-ARDUINO: 2195; DATASHEET: www.yageo.com.tw/exep/pages/download/literatures/PYu-R_INT-thick_7.pdf; DISTRIBUTOR-LINK: https://www.digikey.com/product-detail/en/yageo/RC0402FR-07390RL/311-390LRCT-ND/2827929; DISTRIBUTOR-PN: 311-390LRCT-ND; MANUFACTURER: Yageo; MANUFACTURER-PN: RC0402FR-07390RL; NOTE: NO
R28 = Arduino-rcl:R: SMD Resistor; CODE-ARDUINO: A5559; DATASHEET: http://www.vishay.com/docs/20035/dcrcwe3.pdf; DISTRIBUTOR-LINK: https://www.digikey.com/product-detail/en/vishay-dale/CRCW0402220RFKED/541-220LCT-ND/1183045; DISTRIBUTOR-PN: 541-220LCT-ND; MANUFACTURER: Vishay; MANUFACTURER-PN: CRCW0402220RFKED; NOTE: NO
R30 = Arduino-rcl:R: SMD Resistor; CODE-ARDUINO: 2197; DATASHEET: www.yageo.com.tw/exep/pages/download/literatures/PYu-R_INT-thick_7.pdf; DISTRIBUTOR-LINK: https://www.digikey.com/product-detail/en/yageo/RC0402FR-075K49L/311-5.49KLRCT-ND/729573; DISTRIBUTOR-PN: 311-5.49KLRCT-ND; MANUFACTURER: Yageo; MANUFACTURER-PN: RC0402FR-075K49L; NOTE: NO
R33 = Arduino-rcl:R: SMD Resistor; CODE-ARDUINO: 0233; DATASHEET: http://www.yageo.com/exep/pages/download/literatures/PYu-R_Marking_2.pdf; DISTRIBUTOR-LINK: https://www.digikey.com/product-detail/en/yageo/RC0603JR-070RL/311-0.0GRCT-ND/729622; DISTRIBUTOR-PN: 311-0.0GRCT-ND; MANUFACTURER: Yageo; MANUFACTURER-PN: RC0603JR-070RL; NOTE: NO; PN-ALTERNATIVE1: -
SIM1 = Arduino-connectors:SIM: SIM connector; DATASHEET: http://www.te.com/commerce/DocumentDelivery/DDEController?Action=srchrtrv&DocNm=2199337&DocType=Customer+Drawing&DocLang=English; DISTRIBUTOR-LINK: https://www.digikey.com/product-detail/en/te-connectivity-amp-connectors/2199337-5/A125065CT-ND/6810766; DISTRIBUTOR-PN: A125065CT-ND; MANUFACTURER: TE; MANUFACTURER-PN: 2199337-5
U1 = Arduino-ucs&SoCs:ATSAMD21G18A-48: ARM® Cortex®-M0+ SAM D21G Microcontroller IC 32-Bit 48MHz 256KB (256K x 8) FLASH 48-TQFP (7x7); DATASHEET: http://www.atmel.com/Images/Atmel-42181-SAM-D21_Datasheet.pdf; DISTRIBUTOR-LINK: http://www.digikey.com/product-detail/en/atmel/ATSAMD21G18A-AUT/ATSAMD21G18A-AUTCT-ND/4878879; DISTRIBUTOR-PN: ATSAMD21G18A-AUTCT-ND; MANUFACTURER: Atmel; MANUFACTURER-PN: ATSAMD21G18A-MU
U2 U7 = Arduino-ICs:SN74AVC4T774; DATASHEET: http://www.ti.com/lit/ds/sces693d/sces693d.pdf; DISTRIBUTOR-LINK: https://www.digikey.com/product-detail/en/texas-instruments/SN74AVC4T774RSVR/296-24741-1-ND/2092563; DISTRIBUTOR-PN: 296-24741-1-ND; MANUFACTURER: Texas Instruments; MANUFACTURER-PN: SN74AVC4T774RSVR
U3 = Arduino-ucs&SoCs:SARA-U2: SARA-U2: 3.75G HSPA Cellular Module u-blox.com; DATASHEET: https://www.u-blox.com/sites/default/files/SARA-G3-U2_SysIntegrManual_%28UBX-13000995%29.pdf; DISTRIBUTOR-LINK: https://www.digikey.com/product-detail/en/u-blox-america-inc/SARA-U201/672-1021-1-ND/6150684; DISTRIBUTOR-PN: 672-1021-1-ND; MANUFACTURER: Ublocks; MANUFACTURER-PN: SARA-U201
U4 = Arduino-ICs:ATECC508A-MAHDA-T: Secure authentication and product validation device, EEPROM, I2C, 2.0 - 5.5V; DATASHEET: http://www.atmel.com/Images/Atmel-8923S-CryptoAuth-ATECC508A-Datasheet-Summary.pdf; DISTRIBUTOR-LINK: http://www.digikey.com/product-detail/en/atmel/ATECC508A-MAHDA-T/ATECC508A-MAHDA-TCT-ND/5213071; DISTRIBUTOR-PN: ATECC508A-MAHDA-TCT-ND; MANUFACTURER: Atmel; MANUFACTURER-PN: ATECC508A-MAHDA-T
U5 = Arduino-ICs:BQ24195: IC CHRG MGMT LI-ION/POL; DATASHEET: http://www.ti.com/lit/ds/symlink/bq24195.pdf; DISTRIBUTOR-LINK: https://www.digikey.com/product-detail/en/texas-instruments/BQ24195LRGET/296-35047-1-ND/3725759; DISTRIBUTOR-PN: 296-35047-1-ND; MANUFACTURER: Texas Instruments; MANUFACTURER-PN: BQ24195LRGET
U6 = Arduino-ICs:AP7215-33YG: Linear Voltage Regulator IC Positive Fixed 1 Output 3.3V 600mA SOT-89-3; DATASHEET: http://www.diodes.com/_files/datasheets/AP7215.pdf; DISTRIBUTOR-LINK: http://www.digikey.com/product-search/en?keywords=AP7215-33YG-13DICT-ND%20; DISTRIBUTOR-PN: AP7215-33YG-13DICT-ND; MANUFACTURER: Diodes Incorporated; MANUFACTURER-PN: AP7215-33YG-13
Y1 = Arduino-crystals:32.768KHZ: LF crystal; DATASHEET: http://www.abracon.com/Resonators/ABS07.pdf; DISTRIBUTOR-LINK: http://www.digikey.com/product-detail/en/abracon-llc/ABS07-32.768KHZ-T/535-9542-1-ND/1237009; DISTRIBUTOR-PN: 535-9542-1-ND; MANUFACTURER: Abracon LLC; MANUFACTURER-PN: ABS07-32.768KHZ-T

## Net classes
0 default: width 0.19 mm, drill 0.19 mm
1 usb: width 0.19 mm, drill 0.19 mm, clearance 0.127 mm

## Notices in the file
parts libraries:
Arduino-ucs: Copyright (c) 2016-2017 Arduino LLC. All right reserved.
